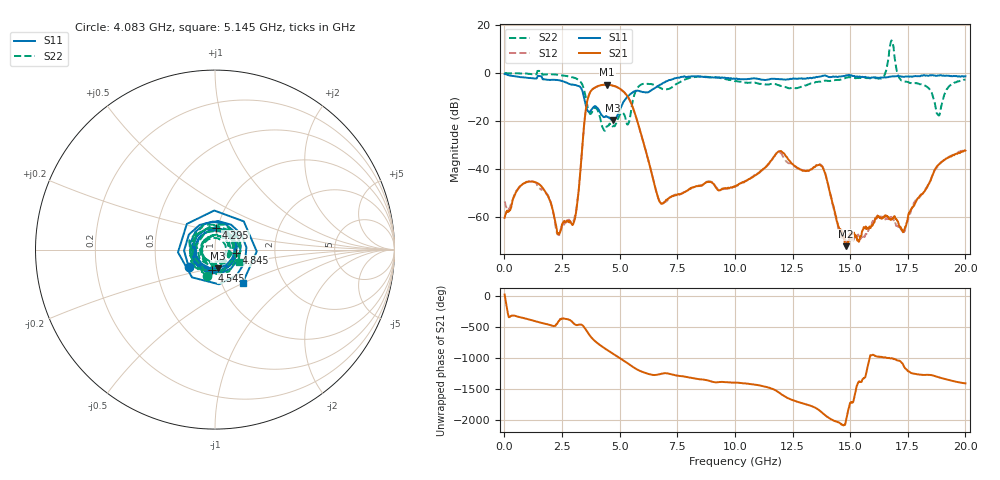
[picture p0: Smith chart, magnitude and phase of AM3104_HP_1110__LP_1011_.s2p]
!Created with skrf (http://scikit-rf.org).
# Hz S RI R 50.0
!freq ReS11 ImS11 ReS21 ImS21 ReS12 ImS12 ReS22 ImS22
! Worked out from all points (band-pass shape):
!   1601 points, 10 MHz to 20 GHz, reference 50 ohm
!   highest |S21| = -4.86 dB at 4.458 GHz (marker M1); lowest = -72.0 dB at 14.82 GHz (marker M2)
!   |S21| within 3 dB of the highest: 3.727 GHz to 5.187 GHz (1.46 GHz wide, 32.8 % of centre)
!   lowest |S11| = -19.6 dB at 4.708 GHz (marker M3), VSWR 1.24, Z = 50.8 - j10.6 ohm
!   |S11| at or under -10 dB: 3.449 GHz to 5.319 GHz (1.87 GHz wide, 42.6 % of centre)
!   |S22| runs from -24.1 to 13.5 dB; largest |S21 - S12| = 0.049
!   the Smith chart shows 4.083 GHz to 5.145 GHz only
!   S11 on the Smith chart (normalised r, x): 4.083 GHz: 0.73, -0.14; 4.295 GHz: 0.99, +0.24; 4.545 GHz: 0.94, -0.22; 4.845 GHz: 1.26, -0.05; 5.145 GHz: 1.26, -0.49
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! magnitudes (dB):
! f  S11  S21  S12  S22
! 10 MHz  -0.4  -60.2  -53.3  0.0
! 1.334 GHz  -2.3  -45.4  -45.4  -0.5
! 2.359 GHz  -3.0  -67.0  -67.2  -0.8
! 3.033 GHz  -5.0  -61.5  -60.3  -2.0
! 3.346 GHz  -6.6  -34.8  -34.8  -4.2
! 3.621 GHz  -15.8  -10.6  -10.7  -14.6
! 4.083 GHz  -15.1  -5.3  -5.4  -16.4
! 4.295 GHz  -18.3  -4.9  -4.9  -23.3
! 4.458 GHz  -18.3  -4.9  -4.9  -22.2
! 4.545 GHz  -18.6  -5.0  -5.1  -21.4
! 4.708 GHz  -19.6  -5.2  -5.3  -22.2
! 4.845 GHz  -18.7  -5.7  -5.7  -20.9
! 5.145 GHz  -12.4  -7.5  -7.5  -16.5
! 6.682 GHz  -5.3  -52.2  -52.3  -5.7
! 10.01 GHz  -2.5  -47.3  -47.2  -3.4
! 11.93 GHz  -2.5  -32.5  -32.8  -5.2
! 13.34 GHz  -2.1  -40.0  -39.9  -4.3
! 14.82 GHz  -1.0  -72.0  -70.6  -2.0
! 16.68 GHz  -1.6  -60.3  -60.3  7.1
! 17.34 GHz  -1.6  -65.2  -65.9  -3.5
! 18.81 GHz  -1.0  -38.3  -38.7  -17.4
! 20 GHz  -1.4  -32.3  -31.9  -2.7
